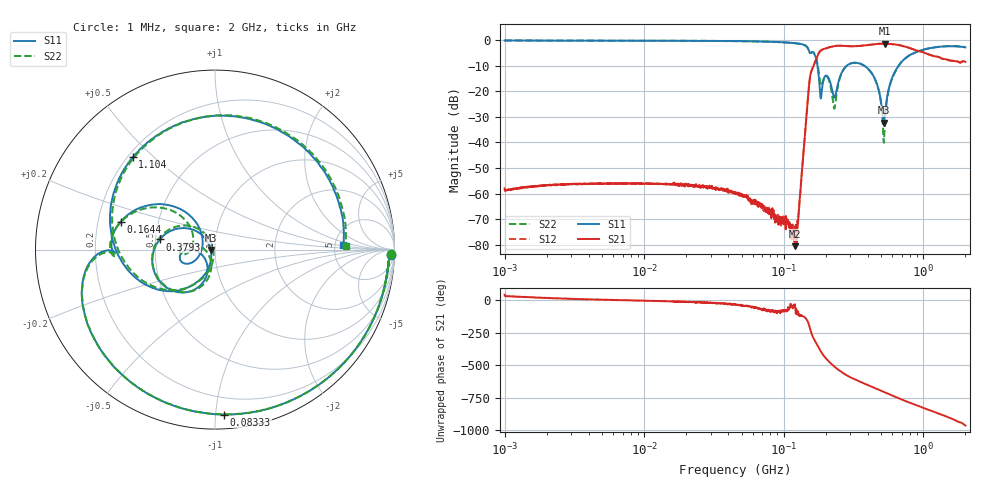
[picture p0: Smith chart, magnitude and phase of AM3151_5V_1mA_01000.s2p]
! Date/Time: Fri Jun 26 10:49:26 2020
! Network Analyzer:  Rev:
! Sweep from 1000000.0 to 2000000000.0, 1601 Points ! Power Supply: 0 V, 0 A
# HZ S DB R 50
!freq MagS11 AngS11 MagS21 AngS21 MagS12 AngS12 MagS22 AngS22
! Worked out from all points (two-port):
!   1601 points, 1 MHz to 2 GHz, reference 50 ohm
!   highest |S21| = -1.42 dB at 531.4 MHz (marker M1); lowest = -80.5 dB at 120.7 MHz (marker M2)
!   |S21| within 3 dB of the highest: 181.9 MHz to 948.3 MHz (766.4 MHz wide, 136 % of centre)
!   lowest |S11| = -32.2 dB at 518.9 MHz (marker M3), VSWR 1.05, Z = 47.6 - j0.18 ohm
!   |S11| at or under -10 dB: 174.2 MHz to 282.7 MHz (108.5 MHz wide, 47.5 % of centre); 376.6 MHz to 664.6 MHz (287.9 MHz wide, 55.3 % of centre)
!   |S22| runs from -40.1 to -0.2 dB; largest |S21 - S12| = 0.0088
!   S11 on the Smith chart (normalised r, x): 1 MHz: 34, -44; 83.33 MHz: 0.09, -1.05; 164.4 MHz: 0.30, +0.13; 379.3 MHz: 0.53, +0.07; 1.104 GHz: 0.22, +0.43; 2 GHz: 5.98, +0.61
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1000000  -0.19 -1.6  -57.90 45.0  -58.49 34.1  -0.19 -1.6
3555161  -0.27 -4.1  -56.24 9.6  -56.15 8.9  -0.26 -4.1
1.263916e7  -0.29 -13.4  -56.11 -4.1  -56.20 -4.7  -0.29 -13.4
4.493426e7  -0.43 -47.1  -60.18 -35.0  -59.88 -30.8  -0.43 -47.1
8.33271e7  -0.72 -86.8  -67.09 -72.9  -67.89 -81.6  -0.74 -86.7
1.207011e8  -1.26 -128.6  -80.47 -48.6  -75.21 -47.2  -1.26 -128.6
1.277818e8  -1.43 -137.9  -67.94 -115.3  -67.20 -107.2  -1.43 -137.7
1.589914e8  -4.77 178.1  -11.62 95.8  -11.61 95.7  -4.72 -179.3
1.643674e8  -5.21 163.5  -9.74 62.1  -9.74 62.1  -5.01 167.0
1.816107e8  -19.98 135.2  -4.45 -22.5  -4.47 -22.5  -15.99 142.7
2.06465e8  -14.27 -172.1  -3.02 -102.8  -3.02 -102.8  -14.72 173.9
2.303028e8  -22.50 -146.1  -2.37 -150.8  -2.37 -150.9  -26.84 -147.1
2.544631e8  -13.94 -110.5  -2.26 172.8  -2.26 172.7  -14.22 -107.0
3.792528e8  -10.08 169.6  -2.12 77.1  -2.15 77.1  -10.15 166.2
4.63e8  -16.91 135.0  -1.56 37.6  -1.58 37.6  -16.98 127.6
5.189154e8  -32.23 -175.6  -1.43 14.6  -1.43 14.5  -39.50 165.6
5.313877e8  -28.65 -124.8  -1.42 9.7  -1.43 9.8  -31.05 -105.9
5.652395e8  -19.04 -109.3  -1.51 -2.9  -1.48 -3.0  -19.37 -104.3
7.660793e8  -6.56 -160.6  -2.82 -62.4  -2.84 -62.4  -6.62 -162.6
1.104424e9  -3.23 131.6  -5.73 -126.5  -5.73 -126.6  -3.23 128.5
1.482693e9  -2.47 73.3  -7.76 -179.1  -7.63 -179.5  -2.40 70.5
2e9  -2.90 2.0  -8.54 114.8  -8.69 114.3  -2.76 1.6
